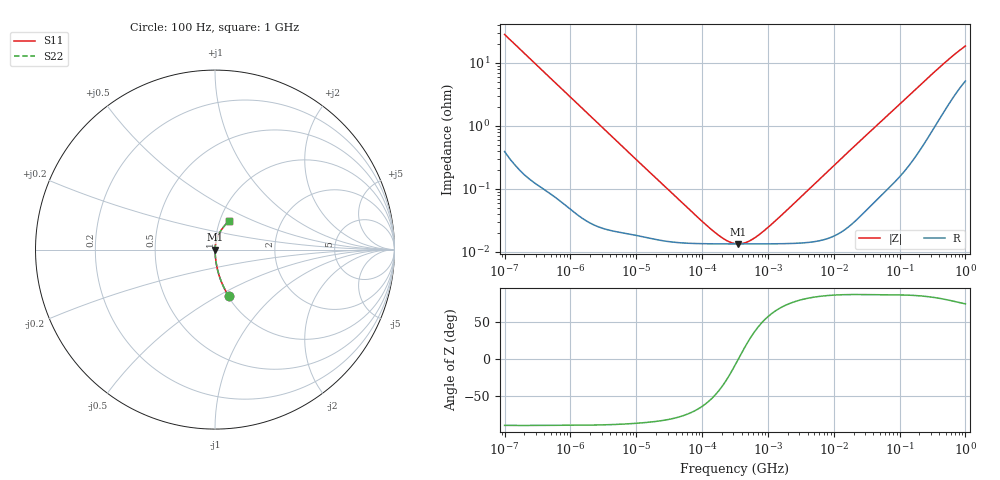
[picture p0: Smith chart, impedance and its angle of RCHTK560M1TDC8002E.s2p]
! RCHTK560M1TDC8002E  S-PARAMETER MODEL  (AEC-Q200 qualified)
! Model Generated by ELNA Corporation (http://www.ty-top.com)
! Version 1.0
! ELNA Control No. 240315
! Copyright (c) 2024 ELNA CO.,LTD. All Rights Reserved.
! Products Name : CONDUCTIVE POLYMER HYBRID ALUMINUM ELECTROLYTIC CAPACITORS
! Characteristics :
!  Capacitance  :  56uF  ,  Rated voltage  :  25V
!  Operating Temp. Range  :  -55 to +125 degC  ,  Endurance  :  4000hr at 125 degC
!  Dimension D  :  6.3mm  ,  Dimension L  :  5.8mm
! Frequency Range : 100Hz - 1GHz
! External Node Assignments :
!  1  o---| |---o  2
# MHz S RI R 50
!Freq[MHz].  S11 Real  S11 Imag  S21 Real  S21 Imag  S12 Real  S12 Imag  S22 Real  S22 Imag
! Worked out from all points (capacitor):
!   401 points, 100 Hz to 1 GHz, reference 50 ohm
!   read as one part in series: C = 56.1 uF near 108 Hz
!   lowest |Z| = 13.4 mohm at 356.9 kHz (marker M1)
!   series resonance near 356.8 kHz, so ESL is about 3.5 nH
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0.0001  0.0775 -0.2605  0.9225 0.2605  0.9225 0.2605  0.0775 -0.2605
0.000113  0.0621 -0.2349  0.9379 0.2349  0.9379 0.2349  0.0621 -0.2349
0.000183  0.0252 -0.1509  0.9748 0.1509  0.9748 0.1509  0.0252 -0.1509
0.000309  0.00954 -0.091  0.9905 0.091  0.9905 0.091  0.00954 -0.091
0.000613  0.00288 -0.0465  0.9971 0.0465  0.9971 0.0465  0.00288 -0.0465
0.001488  0.00072 -0.0193  0.9993 0.0193  0.9993 0.0193  0.00072 -0.0193
0.022131  0.000156 -0.00133  0.9998 0.00133  0.9998 0.00133  0.000156 -0.00133
0.080353  0.000136 -0.000352  0.9999 0.000352  0.9999 0.000352  0.000136 -0.000352
0.147062  0.000135 -0.000168  0.9999 0.000168  0.9999 0.000168  0.000135 -0.000168
0.229087  0.000134 -7.65e-05  0.9999 7.65e-05  0.9999 7.65e-05  0.000134 -7.65e-05
0.316228  0.000134 -2.02e-05  0.9999 2.02e-05  0.9999 2.02e-05  0.000134 -2.02e-05
0.356862  0.000134 4.4e-08  0.9999 -4.4e-08  0.9999 -4.4e-08  0.000134 4.4e-08
0.419276  0.000134 2.71e-05  0.9999 -2.71e-05  0.9999 -2.71e-05  0.000134 2.71e-05
0.512861  0.000134 6.2e-05  0.9999 -6.2e-05  0.9999 -6.2e-05  0.000134 6.2e-05
0.767361  0.000134 0.000141  0.9999 -0.000141  0.9999 -0.000141  0.000134 0.000141
1.40443  0.000135 0.000308  0.9999 -0.000308  0.9999 -0.000308  0.000135 0.000308
4.704354  0.000145 0.00109  0.9999 -0.00109  0.9999 -0.00109  0.000145 0.00109
69.9842  0.0013 0.0155  0.9987 -0.0155  0.9987 -0.0155  0.0013 0.0155
184.0772  0.00507 0.0395  0.9949 -0.0395  0.9949 -0.0395  0.00507 0.0395
412.0975  0.0202 0.083  0.9798 -0.083  0.9798 -0.083  0.0202 0.083
695.825  0.0467 0.125  0.9533 -0.125  0.9533 -0.125  0.0467 0.125
1000  0.0758 0.157  0.9242 -0.157  0.9242 -0.157  0.0758 0.157
